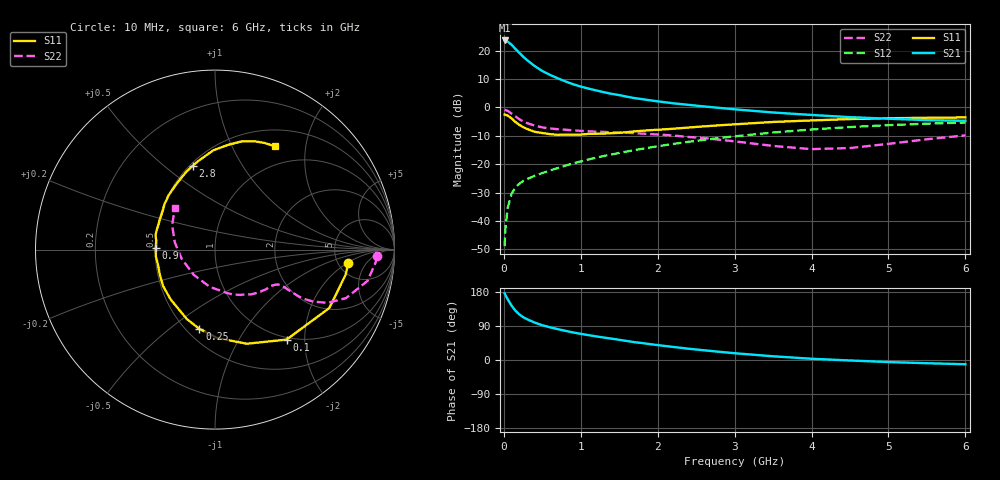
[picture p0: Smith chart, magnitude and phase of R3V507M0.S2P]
! SIEMENS Small Signal Semiconductors
! BFR181
! Si NPN RF Bipolar Junction Transistor in SOT23
! VCE = 0.5 V  IC = 7 mA
! Common Emitter S-Parameters:  May  1996
# GHz  S  MA  R  50
!  f  S11  S21  S12  S22
! GHz  MAG  ANG  MAG  ANG  MAG  ANG  MAG  ANG
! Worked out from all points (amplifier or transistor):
!   36 points, 10 MHz to 6 GHz, reference 50 ohm
!   highest |S21| = 23.6 dB at 10 MHz (marker M1)
!   |S21| within 3 dB of that: start of sweep to 152.1 MHz
!   unconditionally stable (mu >= 1): 374.3 MHz to end of sweep
!   at 250 MHz: K = 0.77, MSG = 21.9 dB, |S12| = -26.0 dB
!   at 1.4 GHz: K = 1.48, MAG = 6.6 dB, |S12| = -16.6 dB
!   at 6 GHz: K = 1.16, MAG = -2.1 dB, |S12| = -5.3 dB
!   S11 on the Smith chart (normalised r, x): 10 MHz: 6.13, -2.13; 100 MHz: 0.96, -1.64; 250 MHz: 0.58, -0.64; 900 MHz: 0.50, +0.01; 2.8 GHz: 0.52, +0.63; 6 GHz: 0.72, +1.48
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0.01  0.7465 -5.9  15.05 175.9  0.0036 83.5  0.9047 -2.4
0.02  0.7409 -11.0  14.85 171.8  0.0071 81.3  0.8966 -4.8
0.05  0.7151 -27.1  14.38 160.2  0.017 76.2  0.8674 -11.6
0.1  0.6406 -51.5  12.66 143.5  0.0299 65.7  0.7785 -20.3
0.15  0.5538 -71.3  10.73 130.2  0.0391 58.5  0.6937 -25.3
0.2  0.4936 -88.2  9.128 120.6  0.0451 54.8  0.6196 -27.9
0.25  0.4504 -101.1  7.816 113.2  0.0503 53.3  0.5647 -29.0
0.3  0.4177 -112.0  6.811 107.7  0.0545 52.5  0.5302 -29.2
0.4  0.3718 -131.6  5.344 98.8  0.0623 53.0  0.4773 -28.9
0.5  0.3535 -144.9  4.361 91.7  0.0696 54.2  0.4437 -28.5
0.6  0.3378 -155.6  3.73 86.3  0.0777 55.6  0.425 -28.4
0.7  0.3286 -165.2  3.25 81.4  0.0852 56.7  0.4129 -28.5
0.9  0.3299 178.7  2.552 72.7  0.1029 58.5  0.394 -29.6
1.1  0.3414 166.2  2.138 65.6  0.1209 59.2  0.3791 -31.8
1.4  0.351 150.9  1.73 56.3  0.1481 59.1  0.3641 -35.8
1.7  0.3782 138.3  1.454 47.0  0.1765 58.3  0.3513 -40.3
2.2  0.4202 121.6  1.18 34.5  0.2269 55.1  0.3201 -51.2
2.8  0.4831 104.9  0.98 21.7  0.2893 49.6  0.2695 -68.1
3.5  0.5535 90.9  0.812 9.8  0.3606 41.5  0.2093 -98.3
4.5  0.6221 75.9  0.672 -1.3  0.45 27.9  0.1923 -164.3
5.5  0.6555 64.9  0.596 -8.5  0.5162 14.6  0.2744 150.5
6  0.665 59.9  0.581 -11.2  0.541 7.7  0.3213 134.2
